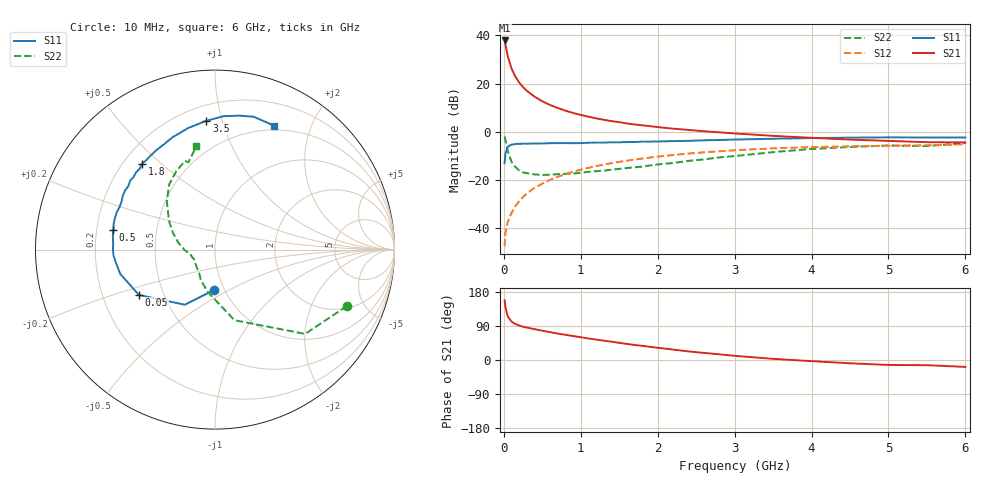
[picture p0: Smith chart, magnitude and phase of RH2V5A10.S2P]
! SIEMENS Small Signal Semiconductors
! BFR106
! Si NPN RF Bipolar Junction Transistor in SOT23
! VCE = 2.5 V  IC = 100 mA
! Common Emitter S-Parameters:  August  1996
# GHz  S  MA  R  50
!  f  S11  S21  S12  S22
! GHz  MAG  ANG  MAG  ANG  MAG  ANG  MAG  ANG
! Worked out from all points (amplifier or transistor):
!   36 points, 10 MHz to 6 GHz, reference 50 ohm
!   highest |S21| = 37.9 dB at 10 MHz (marker M1)
!   |S21| within 3 dB of that: start of sweep to 29.01 MHz
!   unconditionally stable (mu >= 1): 131.7 MHz to 2.988 GHz; 4.635 GHz to end of sweep
!   at 250 MHz: K = 1.10, MAG = 20.8 dB, |S12| = -27.0 dB
!   at 1.4 GHz: K = 1.09, MAG = 6.9 dB, |S12| = -13.0 dB
!   at 6 GHz: K = 1.02, MAG = -0.4 dB, |S12| = -5.1 dB
!   S11 on the Smith chart (normalised r, x): 10 MHz: 0.90, -0.42; 50 MHz: 0.36, -0.24; 500 MHz: 0.27, +0.09; 1.8 GHz: 0.27, +0.43; 3.5 GHz: 0.30, +0.89; 6 GHz: 0.45, +1.49
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0.01  0.2246 -90.9  78.09 157.4  0.0043 72.8  0.7997 -23.2
0.02  0.3501 -118.7  65.43 140.5  0.0078 63.4  0.6874 -43.1
0.05  0.4937 -149.2  37.33 115.6  0.0136 60.9  0.4081 -74.6
0.1  0.5452 -165.7  20.43 101.5  0.021 65.5  0.2405 -99.4
0.15  0.5584 -173.2  13.89 94.8  0.0291 68.9  0.188 -114.8
0.2  0.5667 -176.9  10.54 91.0  0.0368 72.1  0.1585 -123.6
0.25  0.5687 179.3  8.419 87.8  0.0447 72.9  0.1447 -133.0
0.3  0.5679 177.5  7.06 85.5  0.0531 73.8  0.1395 -138.2
0.4  0.5741 172.5  5.354 81.3  0.0694 73.8  0.1315 -147.5
0.5  0.5769 169.2  4.296 77.4  0.0848 73.1  0.1282 -153.6
0.6  0.5824 165.7  3.607 73.5  0.1014 72.4  0.1294 -157.1
0.7  0.5846 162.1  3.124 69.7  0.1174 71.2  0.1331 -160.6
0.9  0.5824 156.0  2.464 63.2  0.1493 68.2  0.1371 -167.2
1.1  0.5956 149.5  2.061 56.8  0.1801 65.2  0.1488 -171.3
1.4  0.6092 141.0  1.669 48.3  0.2248 60.1  0.1642 -177.9
1.8  0.6285 130.4  1.368 37.4  0.2805 53.4  0.1911 172.9
2.2  0.6429 120.7  1.166 27.5  0.3316 46.5  0.2268 163.5
3  0.6933 102.6  0.928 11.0  0.4156 33.0  0.3153 145.1
3.5  0.7194 93.8  0.827 3.1  0.456 25.2  0.3802 134.9
4.5  0.7581 79.9  0.692 -8.7  0.5016 10.8  0.4867 116.4
5.5  0.7652 68.3  0.612 -13.7  0.5265 1.9  0.5078 107.0
6  0.7648 64.5  0.605 -18.2  0.5548 -4.9  0.5852 100.2
